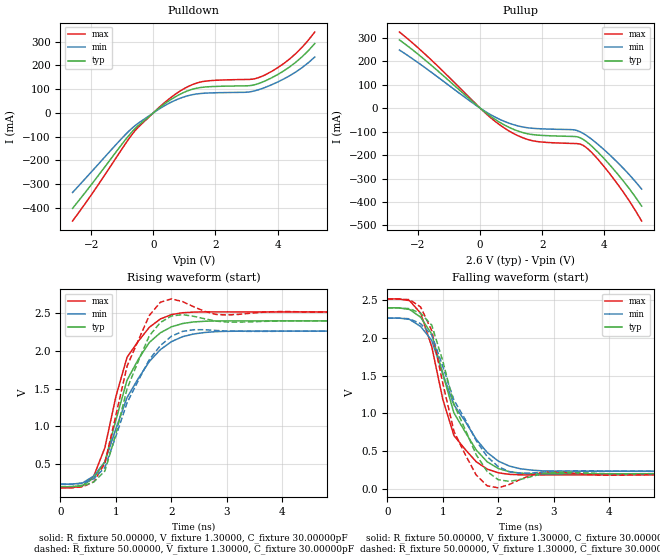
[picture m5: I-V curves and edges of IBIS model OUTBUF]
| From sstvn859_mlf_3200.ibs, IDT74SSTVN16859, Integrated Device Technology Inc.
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|   Model OUTBUF
[Model]   OUTBUF
Model_type   Output
Polarity   Inverting
Vmeas =  1.30000V
Cref = 30.00000pF
Rref =  50.00000
Vref =  1.30000V
C_comp   3.50000pF   3.50000pF   3.50000pF
[Temperature Range]   25.00000   70.00000   0.000
[Voltage Range]   2.60000V   2.50000V   2.70000V
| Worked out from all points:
|   slope of the pulldown table from 0 to 0.39 V, typ, clamps not added: 9.64 ohm
|   slope of the pullup table from 0 to 0.39 V, typ, clamps not added: 9.79 ohm
|   rising waveform, R_fixture 50.00000, V_fixture 1.30000, C_fixture 30.00000pF: 20-80 % time 626ps typ, 749ps min, 562ps max; typ from 0.202 V to 2.4 V
|   rising waveform, R_fixture 50.00000, V_fixture 1.30000, C_fixture 30.00000pF: 20-80 % time 563ps typ, 691ps min, 504ps max; typ from 0.204 V to 2.39 V
|   falling waveform, R_fixture 50.00000, V_fixture 1.30000, C_fixture 30.00000pF: 20-80 % time 663ps typ, 772ps min, 535ps max; typ from 2.4 V to 0.202 V
|   falling waveform, R_fixture 50.00000, V_fixture 1.30000, C_fixture 30.00000pF: 20-80 % time 600ps typ, 713ps min, 459ps max; typ from 2.39 V to 0.204 V
[Pulldown]
| voltage   I(typ)   I(min)   I(max)
-2.6V     -401.8mA   -335.1mA   -455.1mA
-1.8V     -268.7mA   -220.3mA   -307.6mA
-1V       -130mA     -105.2mA   -149.9mA
-600mV    -67.49mA   -54.84mA   -76.8mA
500mV     50.5mA     40.02mA    58.04mA
1V        87.18mA    67.84mA    102.6mA
1.5V      106.4mA    81.32mA    129.3mA
3.1V      114.6mA    88.34mA    141mA
3.6V      134.4mA    107.1mA    160mA
4.4V      194.5mA    157.1mA    227.9mA
4.8V      237.2mA    191.4mA    277.4mA
5.2V      291.9mA    235.2mA    340.4mA
[Pullup]
| voltage   I(typ)   I(min)   I(max)
-2.6V     291.1mA    247.9mA    324.7mA
-1.6V     185.9mA    155.8mA    208.8mA
0V        -2.777nA   -2.095nA   -2.207nA
900mV     -79.93mA   -62.64mA   -94.98mA
1.7V      -112.9mA   -85.98mA   -139.3mA
3V        -120.6mA   -92.11mA   -150.6mA
3.2V      -125.1mA   -99.61mA   -152.5mA
3.4V      -140.7mA   -114.5mA   -166.2mA
3.8V      -188.5mA   -155mA     -219.1mA
4.2V      -245.7mA   -202.7mA   -284.2mA
4.8V      -342.9mA   -283.3mA   -395.1mA
5.2V      -417.8mA   -345mA     -481.3mA
[Ramp]
| variable   typ   min   max
dV/dt_r   1.30200/0.16320n   1.19520/0.19481n   1.38720/0.12588n
dV/dt_f   1.30626/0.15532n   1.20012/0.19309n   1.38660/0.14172n
R_load = 50.00000
[Rising Waveform]
R_fixture = 50.00000
V_fixture = 1.30000
V_fixture_min = 1.25000
V_fixture_max = 1.35000
C_fixture = 30.00000pF
| time   V(typ)   V(min)   V(max)
0s        202.5mV    235.9mV    188mV
400ps     221.7mV    253.5mV    213.5mV
600ps     316.9mV    344.3mV    342.8mV
800ps     531.1mV    531.3mV    717.9mV
1ns       1.087V     971.4mV    1.398V
1.2ns     1.612V     1.382V     1.915V
1.6ns     2.109V     1.857V     2.309V
2ns       2.317V     2.121V     2.478V
3ns       2.395V     2.257V     2.514V
10ns      2.395V     2.26V      2.513V
[Rising Waveform]
R_fixture = 50.00000
V_fixture = 1.30000
V_fixture_min = 1.25000
V_fixture_max = 1.35000
C_fixture = 30.00000pF
R_dut = 0.11300
L_dut = 2.59000nH
C_dut = 0.19900pF
| time   V(typ)   V(min)   V(max)
0s        204.5mV    237.7mV    190.3mV
600ps     264.7mV    308.2mV    268.2mV
800ps     409.3mV    457mV      512.4mV
1.2ns     1.497V     1.312V     1.796V
1.6ns     2.197V     1.881V     2.466V
1.8ns     2.374V     2.068V     2.641V
2ns       2.46V      2.192V     2.686V
2.4ns     2.455V     2.278V     2.582V
3ns       2.38V      2.261V     2.473V
10ns      2.393V     2.258V     2.511V
[Falling Waveform]
R_fixture = 50.00000
V_fixture = 1.30000
V_fixture_min = 1.25000
V_fixture_max = 1.35000
C_fixture = 30.00000pF
| time   V(typ)   V(min)   V(max)
0s        2.395V     2.26V      2.513V
400ps     2.373V     2.242V     2.49V
600ps     2.271V     2.149V     2.324V
800ps     2.047V     1.965V     1.882V
1ns       1.522V     1.521V     1.184V
1.2ns     1.006V     1.112V     707.7mV
1.6ns     517.7mV    660mV      362.2mV
2ns       271.6mV    369.3mV    214.7mV
2.8ns     201.6mV    240.6mV    187mV
10ns      202.5mV    235.9mV    188mV
[Falling Waveform]
R_fixture = 50.00000
V_fixture = 1.30000
V_fixture_min = 1.25000
V_fixture_max = 1.35000
C_fixture = 30.00000pF
R_dut = 0.11300
L_dut = 2.59000nH
C_dut = 0.19900pF
| time   V(typ)   V(min)   V(max)
0s        2.393V     2.258V     2.511V
600ps     2.323V     2.185V     2.406V
800ps     2.167V     2.036V     2.094V
1.2ns     1.119V     1.176V     763.3mV
1.6ns     455.3mV    641.3mV    186.7mV
1.8ns     230.8mV    427.4mV    42.06mV
2ns       122.8mV    295.3mV    16.08mV
2.4ns     126.9mV    209.1mV    129.3mV
3ns       220.9mV    233.3mV    226.6mV
10ns      204.5mV    237.7mV    190.3mV
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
